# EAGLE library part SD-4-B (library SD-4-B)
Memory Card Connectors 11 Positions, Push In, Pull Out, SMT, 2.8 mm Height Above Board, Source: Datasheet
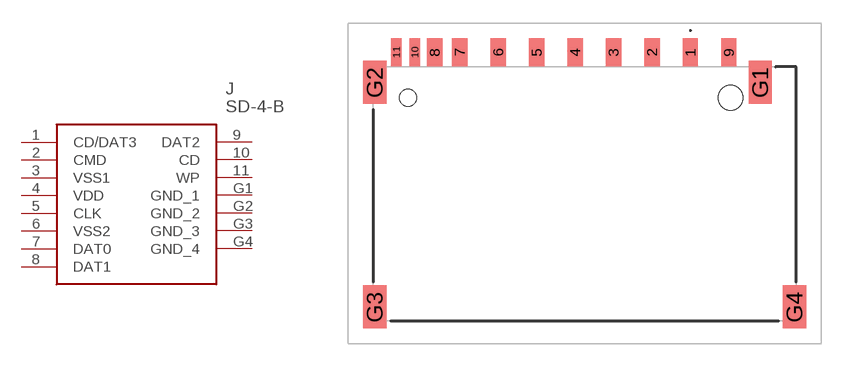
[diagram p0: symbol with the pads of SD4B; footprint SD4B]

Designator prefix J

## SD-4-B (Description: Memory Card Connectors 11 Positions, Push In, Pull Out, SMT, 2.8 mm Height Above Board,; Height: 3.29mm; Manufacturer_Name: CUI Devices; Manufacturer_Part_Number: SD-4-B)  [SD4B]
1  CD/DAT3
2  CMD
3  VSS1
4  VDD
5  CLK
6  VSS2
7  DAT0
8  DAT1
9  DAT2
10  CD
11  WP
G1  GND_1
G2  GND_2
G3  GND_3
G4  GND_4

## Footprint SD4B (pad centres in mm)
SD-4-B-1
smd 1 x 1.8: 1 6.875,8.725; 2 4.375,8.725; 3 1.875,8.725; 4 -0.625,8.725; 5 -3.125,8.725; 6 -5.625,8.725; 7 -8.125,8.725; 8 -9.755,8.725; 9 9.375,8.725
smd 0.7 x 1.8: 10 -11.055,8.725; 11 -12.255,8.725
smd 1.5 x 2.8: G1 11.42,6.775; G2 -13.65,6.775; G3 -13.65,-7.825; G4 13.65,-7.825
hole 1.6 at 9.5,5.775
hole 1.1 at -11.5,5.775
